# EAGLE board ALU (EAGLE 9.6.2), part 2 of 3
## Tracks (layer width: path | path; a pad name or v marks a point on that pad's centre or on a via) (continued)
GND  (via drill 0.35) (continued)
  Bottom 0.152: v64.14,80.96 64.14,76.84 64.77,76.2 C18.2 65.41,76.2 65.41,70.33 63.82,68.74 63.82,66.67 64.45,66.04 C13.2 64.93,65.88 64.93,61.76 v65.38,61.31 65.09,61.02 C43.2 65.41,55.88 65.41,51.44 66.67,50.16 66.67,47.62 64.77,45.72 64.77,44.77 C46.2 65.09,43.5 63.5,41.91 | 64.14,84.45 64.14,87 | 64.14,87 64.14,87.63 C20.2 64.14,87 | 52.23,43.18 52.23,44.29 C27.2 52.07,44.77 48.1,44.77 47.15,43.82 v45.72,43.82 45.72,48.74 43.18,51.28 v43.18,53.34 46.51,53.34 47.62,54.45 48.74,54.45 50.16,55.88 C62.2 | 52.23,43.18 52.23,38.58 | 52.23,38.58 52.23,33.18 C49.2 | 52.23,43.18 58.42,43.18 | 58.42,43.18 59.69,43.18 60.96,41.91 63.5,41.91 | 52.23,38.58 44.45,30.8 v44.45,30.48 | 58.42,43.18 v58.42,42.55 | 65.09,15.24 C47.2 64.77,21.91 64.77,25.56 66.36,27.15 66.36,30.8 65.41,31.75 65.41,33.02 C48.2 65.09,35.24 66.36,36.51 66.36,39.69 64.14,41.91 63.5,41.91 | 51.12,67.95 C14.2 | C19.2 51.44,87.63 51.44,87.15 49.21,87.15 47.78,85.73 47.78,80.8 51.44,77.15 51.44,76.2 C17.2 51.12,75.56 52.07,74.61 52.07,73.66 51.12,72.71 51.12,67.95 | 37.62,60.01 37.62,66.04 C30.2 | 37.47,55.88 37.47,56.99 36.67,57.79 36.67,59.05 37.62,60.01 | 37.62,60.01 41.91,64.29 v41.91,64.45 41.91,66.04 43.81,67.95 51.12,67.95 | C70.2 51.44,8.89 51.44,10.48 49.85,12.07 49.85,15.24 | C69.2 38.73,8.89 38.73,9.84 39.37,10.48 39.37,11.43 43.18,15.24 | 43.18,15.24 49.85,15.24 | 37.47,55.88 37.47,53.02 35.08,50.64 35.08,47.79 C26.2 38.73,44.45 38.73,42.39 40.16,40.96 40.16,38.26 38.73,36.83 38.73,33.02 C53.2 37.91,32.51 v33.91,32.51 33.91,31.81 38.26,27.46 38.26,21.75 C51.2 38.73,21.59 38.73,19.05 v44.45,19.05 43.18,17.78 43.18,15.24
  Bottom 0.152: 37.47,55.88 C9.2 | 49.85,15.24 v56.52,15.24 65.09,15.24 | C44.2 10.48,40.57 11.68,39.37 v15.24,39.37 10.16,34.29 10.16,33.34 C33.2 10.79,33.02 10.79,31.75 12.06,30.48 13.18,30.48 v15.24,28.42 | v27.94,61.59 v27.94,57.15 | v50.48,22.54 50.48,22.38 51.28,21.59 C50.2 52.07,21.59 49.85,19.37 49.85,15.24 | v80.64,71.75 81.6,72.71 83.5,72.71 v84.45,71.75 | 64.14,84.45 65.09,83.5 65.09,81.92 v64.14,80.96 | v57.15,84.45 57.15,84.3 57.94,83.5 63.18,83.5 64.14,84.45 | v80.64,71.75 81.28,71.12 81.28,69.85 80.01,68.58 80.01,66.52 80.49,66.04 | 124.94,33.97 129.22,33.97 v129.54,34.29 | 23.5,57.31 v24.61,57.31 | v68.58,82.55 68.58,82.07 68.08,81.58 64.75,81.58 v64.14,80.96
ITS  (via drill 0.35)
  Top 0.152: v108.74,44.29 108.84,44.29 109.22,43.92 IC67.2 | v121.28,59.05 121.28,57.79 121.92,57.15 IC62.1
  Route2 0.152: v108.74,44.29 108.74,45.24 113.51,50.01 113.51,50.8 121.28,58.58 v121.28,59.05
LDA  (via drill 0.35)
  Top 0.152: v139.7,35.56 IC55.13 | v115.57,46.36 IC67.8 115.57,48.9 115.76,49.08 v115.76,50.29 | IC68.1 107.95,53.98 109.22,55.25 111.76,55.25 112.24,55.72 114.94,55.72 115.41,55.25 116.51,55.25 v116.53,55.22
  Route2 0.152: v139.7,35.56 128.91,46.36 v115.57,46.36
  Route3 0.152: v116.53,55.22 116.53,51.38 115.76,50.61 v115.76,50.29
LDN  (via drill 0.35)
  Top 0.152: IC68.2 109.22,51.44 109.83,50.82 110.76,50.82 111.26,50.32 v112.42,50.32 | v111.76,44.45 112.71,44.45 113.03,44.13 IC67.5 | v131.13,43.18 138.43,43.18 IC56.1
  Route2 0.152: v131.13,43.18 113.03,43.18 v111.76,44.45
  Route3 0.152: v111.76,44.45 111.76,45.4 112.55,46.2 112.55,50.3 112.53,50.32 v112.42,50.32
MA1  (via drill 0.35)
  Top 0.152: v117.47,66.67 118.11,66.04 118.11,60.01 119.38,58.74 119.38,53.98 118.59,53.18 118.59,37.31 v118.11,36.83 | IC69.2 v109.22,66.36 | IC66.11 111.76,36.2 112.55,35.4 114.78,35.4 v114.94,35.56 | v134.94,71.75 133.03,71.75 131.13,69.85 v128.27,69.85 | IC59.1 v138.43,71.75
  Route2 0.152: v109.22,66.36 109.54,66.67 v117.47,66.67 120.65,69.85 122.24,69.85 123.03,70.64 124.3,70.64 125.09,69.85 v128.27,69.85 | v114.94,35.56 116.2,36.83 v118.11,36.83 | v138.43,71.75 v134.94,71.75
MA2  (via drill 0.35)
  Top 0.152: v110.49,50.16 IC67.12 | IC69.6 v114.3,61.59 | v139.7,77.79 IC59.13
  Route3 0.152: v110.49,50.16 110.49,52.71 115.57,57.79 115.57,60.33 v114.3,61.59
  Route14 0.152: v139.7,77.79 139.22,77.79 128.43,66.99 126.68,66.99 125.25,65.56 125.25,64.29 122.56,61.59 v114.3,61.59
MN1  (via drill 0.35)
  Top 0.152: IC66.4 111.76,29.53 v110.33,28.1 | v107.31,60.96 107.63,60.96 107.95,61.28 IC69.1 | v138.43,86.36 IC60.1
  Route3 0.152: v138.43,86.36 138.43,83.19 127.95,72.71 117,72.71 114.04,69.75 113.57,69.75 107.31,63.5 v107.31,60.96
  Bottom 0.152: v110.33,28.1 110.33,30 106.68,33.66 106.68,51.75 106.05,52.39 106.05,55.88 107.31,57.15 v107.31,60.96
MN2  (via drill 0.35)
  Top 0.152: v114.3,65.41 113.03,64.14 IC69.5 | IC60.13 139.7,91.44 139.06,92.08 137.79,92.08 130.18,84.45 130.18,71.12 129.7,70.64 124.62,70.64 v123.19,69.22 | v108.03,41.42 107.95,41.5 IC67.1
  Route2 0.152: v114.3,65.41 v109.86,60.96
  Route3 0.152: v108.03,41.42 107.98,41.47 107.98,59.08 v109.86,60.96
  Bottom 0.152: v114.3,65.41 114.3,66.2 115.89,67.79 116.84,67.79 116.92,67.87 122.79,67.87 123.19,68.26 v123.19,69.22
MUL/IN/T1/N0  (via drill 0.35)
  Top 0.152: IC31.1 49.53,16.83 49.85,16.51 v52.07,16.51 | v63.18,21.91 62.23,20.95 IC32.1 | v81.28,20.32 IC27.4
  Route14 0.152: v81.28,20.32 81.28,22.38 79.85,23.81 65.09,23.81 v63.18,21.91
  Bottom 0.152: v52.07,16.51 56.04,20.48 56.04,21.43 57.47,22.86 62.23,22.86 v63.18,21.91
MUL/IN/T1/N1  (via drill 0.35)
  Top 0.152: v58.26,24.92 57.15,24.92 IC31.8 | v68.58,22.22 69.85,23.49 IC32.8 | v79.38,20.32 79.69,20.32 82.55,23.18 IC27.10
  Route2 0.152: v58.26,24.92 65.88,24.92 v68.58,22.22
  Bottom 0.152: v79.38,20.32 70.48,20.32 v68.58,22.22
MUL/IN/T1/N2  (via drill 0.35)
  Top 0.152: IC35.1 7.62,17.14 9.37,15.4 10.95,15.4 v12.06,16.51 | v20.32,18.41 21.59,18.41 IC34.1 | v79.38,22.86 80.96,22.86 81.28,23.18 IC27.11
  Route2 0.152: v12.06,16.51 12.38,16.19 18.1,16.19 v20.32,18.41
  Route14 0.152: v79.38,22.86 71.28,22.86 69.61,21.19 65.64,21.19 62.87,18.41 47.15,18.41 45.88,17.14 41.27,17.14 40.01,18.41 v20.32,18.41
MUL/IN/T1/N3  (via drill 0.35)
  Top 0.152: v15.24,22.22 IC35.8 | IC34.8 v29.21,22.22
  Route2 0.152: v15.24,22.22 15.72,22.7 27.17,22.7 27.67,22.2 28.21,22.2 28.23,22.22 v29.21,22.22
MUL/IN/T2/N0  (via drill 0.35)
  Top 0.152: v49.85,20.95 50.8,20 IC31.2 | IC32.2 v63.5,20.95 | IC28.3 80.01,29.21 v78.74,27.94
  Route2 0.152: v49.85,20.95 53.98,20.95 55.4,22.38 61.28,22.38 62.71,20.95 v63.5,20.95 68.58,20.95 75.56,27.94 v78.74,27.94
MUL/IN/T2/N1  (via drill 0.35)
  Top 0.152: IC31.9 55.88,23.23 57.47,21.65 v57.47,21.43 | v81.28,31.75 IC28.4 | v68.58,26.04 IC32.9
  Route3 0.152: v81.28,31.75 80.8,31.27 73.82,31.27 v68.58,26.04 65.09,26.04 v60.64,21.59
  Bottom 0.152: v60.64,21.59 60.48,21.43 v57.47,21.43
MUL/IN/T2/N2  (via drill 0.35)
  Top 0.152: IC35.2 8.89,19.68 v9.53,20.32 | v17.14,17.14 22.7,17.14 22.86,17.3 IC34.2 | IC28.10 82.55,34.92 v83.19,34.29
  Route2 0.152: v9.53,20.32 12.7,17.14 v17.14,17.14
  Route15 0.152: v83.19,34.29 81.92,34.29 78.9,31.27 75.72,31.27 62.87,18.41 47.15,18.41 45.88,17.14 v17.14,17.14
MUL/IN/T2/N3  (via drill 0.35)
  Top 0.152: v13.97,22.86 IC35.9 | v27.94,22.86 IC34.9 | v81.44,37.78 81.44,37.68 81.28,37.52 IC28.11
  Route2 0.152: v13.97,22.86 14.45,23.34 27.46,23.34 v27.94,22.86
  Route3 0.152: v81.44,37.78 81.12,37.78 78.26,34.92 71.91,34.92 70.33,33.34 62.39,33.34 61.44,34.29 58.58,34.29 57.47,35.4 51.59,35.4 51.12,34.92 46.35,34.92 41.91,30.48 35.56,30.48 v27.94,22.86
MUL/IN/T3/N0  (via drill 0.35)
  Top 0.152: v50.8,31.75 50.48,31.75 49.53,30.8 IC36.1 | v62.23,27.94 IC37.1 | IC29.3 80.01,40.64 v78.74,39.37
  Route2 0.152: v78.74,39.37 72.87,39.37 62.23,28.73 v62.23,27.94
  Bottom 0.152: v50.8,31.75 57.15,31.75 60.96,27.94 v62.23,27.94
MUL/IN/T3/N1  (via drill 0.35)
  Top 0.152: v58.42,35.56 57.15,35.56 IC36.8 | v70.8,35.56 69.85,35.56 IC37.8 | v78.74,38.1 80.49,39.85 81.12,39.85 81.28,40.01 IC29.4
  Route3 0.152: v70.8,35.56 v58.42,35.56
  Bottom 0.152: v78.74,38.1 73.34,38.1 v70.8,35.56
MUL/IN/T3/N2  (via drill 0.35)
  Top 0.152: IC39.1 21.59,31.11 21.46,31.24 v21.59,31.37 | v7.62,31.43 IC40.1 | IC29.10 82.55,44.45 v81.28,43.18
  Route2 0.152: v7.62,31.43 7.62,27.94 8.26,27.3 11.43,27.3 15.27,31.15 18.07,31.15 18.8,31.88 21.08,31.88 v21.59,31.37
  Route15 0.152: v81.28,43.18 74.93,36.83 48.42,36.83 47.62,37.62 43.66,37.62 42.23,36.2 23.18,36.2 21.59,34.61 v21.59,31.37
MUL/IN/T3/N3  (via drill 0.35)
  Top 0.152: v19.05,35.56 15.24,35.56 IC40.8 | IC39.8 v29.21,34.61 | IC29.11 81.28,45.09 v79.38,43.18
  Route3 0.152: v19.05,35.56 19.3,35.31 28.51,35.31 v29.21,34.61 44.13,34.61 51.12,41.59 69.22,41.59 70.8,43.18 74.45,43.18 75.56,42.07 78.26,42.07 v79.38,43.18
MUL/IN/T4/N0  (via drill 0.35)
  Top 0.152: v49.53,43.82 IC41.1 | IC42.1 v62.23,42.86 | v80.01,54.29 IC30.3
  Route2 0.152: v62.23,42.86 61.59,43.5 52.23,43.5 51.28,44.45 50.16,44.45 v49.53,43.82
  Route14 0.152: v80.01,54.29 72.07,54.29 62.23,44.45 v62.23,42.86
MUL/IN/T4/N1  (via drill 0.35)
  Top 0.152: v58.58,47.47 57.21,47.47 IC41.8 | v69.53,49.21 69.85,48.9 IC42.8 | IC30.4 81.28,51.59 80.8,51.12 v79.85,51.12
  Route2 0.152: v58.58,47.47 67.79,47.47 v69.53,49.21 71.44,51.12 v79.85,51.12
MUL/IN/T4/N2  (via drill 0.35)
  Top 0.152: IC45.1 7.62,40.01 9.21,38.42 18.41,38.42 20,40.01 v21.59,40.01 IC44.1 | v82.55,57.47 IC30.10
  Route2 0.152: v81.28,50.16 81.12,50.32 71.91,50.32 62.23,40.64 41.12,40.64 40.64,41.12 36.2,41.12 35.72,40.64 22.23,40.64 v21.59,40.01
  Route3 0.152: v82.55,57.47 82.55,55.88 81.28,54.61 v81.28,50.16
MUL/IN/T4/N3  (via drill 0.35)
  Top 0.152: v17.78,47.62 15.24,47.62 IC45.8 | v30.48,47.62 29.21,47.62 IC44.8 | v81.28,60.33 IC30.11
  Route2 0.152: v30.48,47.62 v17.78,47.62
  Route3 0.152: v81.28,60.33 79.38,60.33 70.48,51.44 65.88,51.44 64.29,49.85 61.59,49.85 60.01,51.44 52.55,51.44 50.96,49.85 48.42,49.85 46.83,51.44 34.29,51.44 v30.48,47.62
MUL/OUT/N0  (via drill 0.35)
  Top 0.152: IC27.3 80.01,17.14 v80.64,16.51 | IC50.13 v49.53,88.27
  Route2 0.152: v49.53,88.27 50.16,87.63 50.16,85.73 60.96,74.93 60.96,72.07 63.66,69.37 66.52,69.37 70.17,65.72 70.17,62.87 81.92,51.12 82.87,51.12 85.09,48.9 85.09,37.47 82.15,34.53 82.15,18.02 v80.64,16.51
MUL/OUT/N1  (via drill 0.35)
  Top 0.152: IC33.3 38.1,21.59 v39.37,22.86 | IC50.9 v54.61,87.63
  Route14 0.152: v39.37,22.86 39.37,36.83 44.69,42.15 44.69,60.56 54.61,70.48 54.61,74.93 56.2,76.52 56.2,86.04 v54.61,87.63
MUL/OUT/N2  (via drill 0.35)
  Top 0.152: v38.1,31.43 IC38.3 | IC50.6 v54.61,86.04
  Route14 0.152: v38.1,31.43 38.1,34.29 32.38,40.01 32.38,50.64 32.86,51.12 32.86,52.71 32.38,53.18 32.38,57.47 31.75,58.1 31.75,64.45 33.66,66.36 33.66,67.31 43.97,77.63 43.97,79.85 50.16,86.04 v54.61,86.04
MUL/OUT/N3  (via drill 0.35)
  Top 0.152: IC50.2 v49.53,83.19 | IC43.3 v38.1,40.01
  Route14 0.152: v38.1,40.01 38.1,46.04 39.05,46.99 39.05,60.01 49.85,70.8 49.85,76.84 48.1,78.58 48.1,81.76 v49.53,83.19
MUL/OUT/N4  (via drill 0.35)
  Top 0.152: v46.99,48.26 44.29,45.56 41.75,45.56 39.37,43.18 IC43.4 | v87.63,48.26 87.63,61.59 93.98,67.95 IC51.13
  Route15 0.152: v87.63,48.26 83.82,48.26 82.71,47.15 75.09,47.15 73.98,48.26 v46.99,48.26
MUL/OUT/N5  (via drill 0.35)
  Top 0.152: v94.61,64.77 97.16,67.31 98.61,67.31 99.06,67.75 IC51.9 | IC43.10 40.64,49.37 41.43,50.16 44.45,50.16 v46.99,52.71
  Route3 0.152: v46.99,52.71 57.78,52.71 65.25,60.17 66.2,60.17 67.31,61.28 67.31,62.23 68.58,63.5 80.01,63.5 80.64,64.14 93.98,64.14 v94.61,64.77
MUL/OUT/N6  (via drill 0.35)
  Top 0.152: v39.37,45.72 IC43.11 | IC51.6 v99.06,61.47
  Route3 0.152: v39.37,45.72 48.26,45.72 50.64,48.1 56.67,48.1 56.83,48.26 74.77,48.26 75.41,47.62 82.39,47.62 83.82,49.05 91.73,49.05 97.54,54.86 97.54,61.21 97.79,61.47 v99.06,61.47
MUL/OUT/N7  (via drill 0.35)
  Top 0.152: v25.4,48.9 IC44.11 | v88.9,61.59 93.34,61.59 93.98,62.23 IC51.2
  Route3 0.152: v25.4,48.9 27.3,50.8 29.21,50.8 30.8,52.39 46.04,52.39 46.35,52.07 46.63,51.79 48.93,51.79 49.21,52.07 68.58,52.07 77.31,60.8 80.49,60.8 82.23,62.55 87.95,62.55 v88.9,61.59
MUL/OUT/T1/N0  (via drill 0.35)
  Top 0.152: v49.53,26.99 46.99,26.99 45.4,25.4 45.4,23.81 43.18,21.59 40.96,21.59 39.37,20 IC33.4 | IC36.2 v50.8,28.57 | v61.59,31.75 63.18,31.75 63.5,31.43 IC37.2
  Route2 0.152: v49.53,26.99 50.8,28.26 v50.8,28.57
  Route14 0.152: v61.59,31.75 53.98,31.75 v50.8,28.57
MUL/OUT/T1/N1  (via drill 0.35)
  Top 0.152: IC33.10 40.64,26.04 43.18,28.57 46.35,28.57 v50.8,33.02 | IC36.9 v55.88,34.13 | IC37.9 68.58,37.47 67.63,38.42 v65.25,38.42
  Route2 0.152: v50.8,33.02 54.77,33.02 v55.88,34.13
  Bottom 0.152: v65.25,38.42 65.09,38.42 60.64,33.97 56.04,33.97 v55.88,34.13
MUL/OUT/T1/N2  (via drill 0.35)
  Top 0.152: IC39.2 v22.86,28.57 | IC33.11 39.37,25.4 v37.47,27.3 | IC40.2 v8.89,28.57
  Route2 0.152: v37.47,27.3 34.29,27.3 33.02,28.57 28.89,28.57 27.94,29.53 25.72,29.53 24.77,28.57 v22.86,28.57
  Route14 0.152: v22.86,28.57 22.83,28.6 19.37,28.6 17.81,30.16 10.48,30.16 v8.89,28.57
MUL/OUT/T1/N3  (via drill 0.35)
  Top 0.152: IC34.11 v25.4,26.04 | v13.97,34.61 IC40.9 | v27.94,34.61 IC39.9
  Route14 0.152: v13.97,34.61 20.32,34.61 21.27,35.56 26.99,35.56 v27.94,34.61 28.89,33.66 28.89,28.26 26.67,26.04 v25.4,26.04
MUL/OUT/T2/N0  (via drill 0.35)
  Top 0.152: v47.94,33.02 40.96,33.02 39.37,31.43 IC38.4 | IC41.2 v50.8,38.1 | v63.5,40.01 IC42.2
  Route2 0.152: v63.5,40.01 60.33,36.83 57.31,36.83 56.67,36.2 52.7,36.2 v50.8,38.1 50.8,35.88 v47.94,33.02
MUL/OUT/T2/N1  (via drill 0.35)
  Top 0.152: v48.26,46.99 47.62,46.36 47.62,42.23 44.77,39.37 42.23,39.37 40.64,37.78 IC38.10 | IC41.9 v55.88,49.53 | IC42.9 68.58,48.26 66.99,49.85 v65.88,49.85
  Route2 0.152: v48.26,46.99 49.53,48.26 54.61,48.26 v55.88,49.53
  Bottom 0.152: v65.88,49.85 62.71,46.67 58.1,46.67 55.88,48.9 v55.88,49.53
MUL/OUT/T2/N2  (via drill 0.35)
  Top 0.152: v8.89,42.8 IC45.2 | IC44.2 v22.86,38.1 | v39.37,38.73 IC38.11
  Route2 0.152: v8.89,42.8 9.27,42.8 13.97,38.1 21.3,38.1 21.32,38.08 21.86,38.08 21.89,38.1 v22.86,38.1 24.13,39.37 25.88,39.37 26.51,38.73 v39.37,38.73
MUL/OUT/T2/N3  (via drill 0.35)
  Top 0.152: v13.97,46.04 IC45.9 | IC44.9 v27.94,45.09 | IC39.11 25.4,37.08 27.3,38.99 v27.3,39.69
  Route2 0.152: v13.97,46.04 14.95,45.06 16.46,45.06 16.49,45.09 v27.94,45.09
  Route14 0.152: v27.3,39.69 26.19,40.8 26.19,43.34 v27.94,45.09
N$1  (via drill 0.35)
  Top 0.152: v81.92,74.45 IC1.5 | v113.03,81.92 113.03,81.53 112.39,80.9 IC2.12
  Route2 0.152: v81.92,74.45 81.92,77.47 83.82,79.38 86.36,81.92 92.39,81.92 94.3,83.82 99.54,83.82 101.44,81.92 109.08,81.92 109.58,82.41 110.13,82.41 110.63,81.92 v113.03,81.92
N$2  (via drill 0.35)
  Top 0.152: IC7.13 111.12,89.15 109.86,87.88 IC7.3 v109.86,81.76 | v96.52,31.75 IC10.4 | v93.98,44.45 93.98,50.16 94.61,50.8 IC5.3 94.61,53.34 95.89,54.61 IC5.13
  Route3 0.152: v96.52,31.75 96.52,41.91 95.25,43.18 | v93.98,44.45 95.25,43.18 | v109.86,81.76 111.92,81.76 113.19,80.49 115.89,80.49 120.33,76.04 120.33,75.09 118.52,73.28 113.92,73.28 110.49,69.85 108.9,69.85 107.63,68.58 107.63,66.99 100.97,60.33 100.97,48.9 95.25,43.18
N$3  (via drill 0.35)
  Top 0.152: IC1.13 80.64,77.47 79.38,76.2 IC1.3 v79.38,71.75 | IC10.3 95.25,28.89 96.2,27.94 v96.52,27.94 | IC3.3 94.61,43.18 95.89,44.45 IC3.13 v95.89,45.97
  Route14 0.152: v79.38,71.75 79.38,71.12 79.06,70.8 79.06,68.9 89.53,58.42 89.53,52.68 89.72,52.5 89.72,51.16 89.53,50.98 89.53,46.74 | 89.53,46.74 89.53,34.92 91.44,33.02 91.44,31.11 93.19,29.37 94.77,29.37 96.2,27.94 v96.52,27.94 | v89.44,46.74 89.53,46.74
  Route15 0.152: v95.89,45.97 93.98,45.97 93.22,46.74 v89.44,46.74
N$4  (via drill 0.35)
  Top 0.152: v83.19,77.47 IC1.11 | v102.87,78.11 103.35,77.63 108.11,77.63 108.58,78.11 IC2.15
  Route2 0.152: v102.87,78.11 102.71,78.11 101.6,79.22 84.93,79.22 v83.19,77.47
N$5  (via drill 0.35)
  Top 0.152: v100.33,43.18 97.79,43.18 97.16,42.55 IC3.5 | v130.65,27.3 135.1,22.86 135.1,17.94 135.89,17.14 138.75,17.14 139.06,17.46 IC4.2
  Route2 0.152: v100.33,43.18 104.14,43.18 107,40.32 108.9,40.32 109.62,39.61 109.62,38.18 115.65,32.15 117.08,32.15 121.92,27.3 v130.65,27.3
N$6  (via drill 0.35)
  Top 0.152: v89.38,90.81 85.09,90.81 IC6.8 | v102.23,90.81 107.31,85.73 IC7.1
  Route2 0.152: v102.23,90.81 v89.38,90.81
N$7  (via drill 0.35)
  Top 0.152: v82.55,85.88 IC6.5 | IC7.15 108.58,92.08 107.95,92.71 106.68,92.71 v105.25,91.28
  Route3 0.152: v105.25,91.28 103.5,89.53 92.71,89.53 89.06,85.88 v82.55,85.88
N$8  (via drill 0.35)
  Top 0.152: IC3.11 98.42,46.04 98.74,45.72 v99.06,45.72 | v138.43,23.49 141.6,20.32 IC4.4
  Route14 0.152: v99.06,45.72 111.76,45.72 114.46,43.02 122.08,43.02 122.56,42.55 127.48,42.55 128.35,41.67 128.35,36.75 138.43,26.67 v138.43,23.49
N$9  (via drill 0.35)
  Top 0.152: IC5.5 97.16,51.44 v97.79,50.8 | IC2.6 113.67,71.18 v113.32,70.83
  Route14 0.152: v113.32,70.83 111.32,68.83 108.2,68.83 105.06,65.69 v105.06,60.96
  Bottom 0.152: v97.79,50.8 98.42,51.44 104.01,51.44 105.06,52.48 v105.06,60.96
N$10  (via drill 0.35)
  Top 0.152: v92.08,54.61 IC5.1 | IC6.1 v77.47,81.28
  Route14 0.152: v86.36,69.22 86.36,73.03 78.11,81.28 v77.47,81.28
  Bottom 0.152: v92.08,54.61 92.08,63.5 v86.36,69.22
N$11  (via drill 0.35)
  Top 0.152: IC5.15 93.34,57.59 v93.31,57.56 | IC6.12 v80.01,89.22
  Route15 0.152: v80.01,89.22 80.01,84.14 82.23,81.92 v83.19,81.92
  Bottom 0.152: v93.31,57.56 92.88,58 92.88,68.74 92.41,69.21 92.41,71.93 83.19,81.15 v83.19,81.92
N$12  (via drill 0.35)
  Top 0.152: IC2.10 v114.94,75.56 | IC5.11 v98.42,60.45
  Route2 0.152: v114.94,75.56 114.94,74.93 113.86,73.85 111.76,73.85 109.98,72.07 108.9,72.07 v106.68,69.85 | v103.89,67.06 100.58,67.06 97.63,64.1 97.63,61.25 v98.42,60.45
  Route3 0.152: v106.68,69.85 v103.89,67.06
N$13  (via drill 0.35)
  Top 0.152: IC2.2 108.58,74.52 v108.54,74.56 | IC7.5 112.39,82.55 110.49,80.64 108.9,80.64 v108.58,80.96
  Bottom 0.152: v108.58,80.96 108.86,80.69 108.86,74.88 v108.54,74.56
N$14  (via drill 0.35)
  Top 0.152: IC70.5 97.79,17.14 95.89,15.24 v90.17,15.24
  Bottom 0.152: REGISTER/OUT.4 v90.17,15.24
N$15
  Top 0.152: IC26.11 67.94,76.2 68.74,75.41 70.96,75.41 71.75,76.2 71.75,86.68 69.69,88.74 65.25,88.74 64.77,89.22 IC9.11
N$16  (via drill 0.35)
  Top 0.152: IC2.4 111.12,74.3 v111.76,74.93 | v111.92,86.2 111.92,87.15 113.67,88.9 IC7.11
  Bottom 0.152: v111.92,86.2 112.55,85.57 112.55,82.71 111.76,81.92 v111.76,74.93
N$17  (via drill 0.35)
  Top 0.152: v55.24,54.61 53.66,54.61 53.34,54.29 IC16.5 | v64.45,54.45 64.45,54.39 64.77,54.08 IC17.3 64.77,52.07 65.41,51.44 66.67,51.44 67.31,52.07 IC17.5
  Route2 0.152: v55.24,54.61 56.04,55.4 63.5,55.4 v64.45,54.45
N$18  (via drill 0.35)
  Top 0.152: IC18.1 34.29,54.13 33.66,54.77 33.66,55.88 v34.92,57.15 | IC16.3 v50.8,54.29
  Route2 0.152: v50.8,54.29 50.8,53.34 50.16,52.71 48.26,52.71 42.55,58.42 36.2,58.42 v34.92,57.15
N$19  (via drill 0.35)
  Top 0.152: v100.33,22.22 IC70.8
  Route2 0.152: REGISTER/OUT.3 84.45,6.35 95.89,17.78 99.06,17.78 100.33,19.05 v100.33,22.22
N$20  (via drill 0.35)
  Top 0.152: v84.45,65.41 83.5,65.41 82.55,64.45 IC8.5 | v90.81,20.32 v90.81,36.83
  Bottom 0.152: v90.81,36.83 90.81,42.07 90.33,42.55 90.33,44.45 90.81,44.93 90.81,52.07 86.36,56.52 86.36,63.5 v84.45,65.41 | v90.81,20.32 91.6,19.53 91.6,11.59 REGISTER/OUT.2
N$21
  Top 0.152: IC12.5 53.34,4.45 55.88,1.91 63.5,1.91 64.77,3.17 | IC11.3 64.77,3.17 | IC11.5 67.31,4.45 66.04,3.17 64.77,3.17
N$22  (via drill 0.35)
  Top 0.152: v87,36.83 86.84,36.99 86.84,64.93 v87,65.09 | IC8.12 v80.01,70.48
  Route3 0.152: v87,36.83 87,8.26 REGISTER/OUT.1 | v80.01,70.48 81.6,70.48 v87,65.09
N$25
  Top 0.152: IC13.1 35.56,4.13 37.15,2.54 50.16,2.54 50.8,3.17 IC12.3
N$29  (via drill 0.35)
  Top 0.152: IC13.2 v36.83,4.43 | v52.07,4.45 IC12.4
  Route3 0.152: v36.83,4.43 38.4,2.86 50.8,2.86 52.07,4.13 v52.07,4.45
N$30  (via drill 0.35)
  Top 0.152: v45.72,56.52 45.09,55.88 38.1,55.88 35.56,53.34 IC18.2 | v53.98,49.53 53.98,50.16 52.07,52.07 IC16.4
  Route14 0.152: v45.72,56.52 51.44,50.8 52.7,50.8 v53.98,49.53
N$31  (via drill 0.35)
  Top 0.152: v49.53,10.16 IC12.13 | v66.04,4.45 IC11.4 66.04,6.98 63.5,9.53 IC11.13
  Bottom 0.152: v49.53,10.16 49.53,8.26 53.98,3.81 65.41,3.81 v66.04,4.45
N$32  (via drill 0.35)
  Top 0.152: v49.53,57.15 IC16.13 | IC17.13 63.5,56.52 v62.87,56.52 64.14,56.52 66.04,54.61 IC17.4
  Route2 0.152: v49.53,57.15 50.48,56.2 62.55,56.2 v62.87,56.52
N$33  (via drill 0.35)
  Top 0.152: v18.57,55.09 18.41,54.93 17.46,54.93 17.14,54.61 14.61,54.61 13.97,53.98 IC20.6 | IC19.6 v26.67,55.25 | v66.04,57.15 IC17.11
  Route2 0.152: v26.67,55.25 26.04,54.61 19.05,54.61 v18.57,55.09
  Route15 0.152: v66.04,57.15 65.56,57.63 55.72,57.63 55.17,57.07 55.17,56.28 52.39,53.5 47.31,53.5 44.93,55.88 27.3,55.88 v26.67,55.25
N$38  (via drill 0.35)
  Top 0.152: v50.8,60.96 IC16.12 | 64.77,60.64 63.82,60.64 v63.5,60.96 | IC17.12 64.77,60.64 | IC17.10 67.31,60.33 66.99,60.64 64.77,60.64
  Bottom 0.152: v50.8,60.96 51.12,61.28 63.18,61.28 v63.5,60.96
N$39  (via drill 0.35)
  Top 0.152: IC15.6 13.97,3.81 14.76,3.02 v19.68,3.02 | v23.5,3.02 26.19,3.02 27.94,4.76 IC14.6 | v66.04,10.16 IC11.11
  Route2 0.152: v19.68,3.02 v23.5,3.02 23.81,3.33 47.15,3.33 47.94,2.54 59.37,2.54 66.04,9.21 v66.04,10.16
N$40  (via drill 0.35)
  Top 0.152: v50.8,13.34 IC12.12 | IC11.12 64.77,13.65 65.09,13.97 v66.04,13.97 66.99,13.97 67.31,13.65 IC11.10
  Route2 0.152: v50.8,13.34 50.8,12.22 51.28,11.75 63.82,11.75 v66.04,13.97
N$41
  Top 0.152: IC13.5 40.64,7.62 42.07,9.05 51.91,9.05 53.34,10.48 IC12.10
N$42  (via drill 0.35)
  Top 0.152: IC12.11 v52.07,13.34 | v41.91,4.45 IC13.6
  Route3 0.152: v52.07,13.34 50.48,11.75 49.21,11.75 v41.91,4.45
N$43  (via drill 0.35)
  Top 0.152: v48.26,55.25 48.1,55.4 40.16,55.4 39.37,54.61 IC18.5 | v52.07,54.61 52.07,56.2 53.34,57.47 IC16.10
  Route2 0.152: v48.26,55.25 51.44,55.25 v52.07,54.61
N$44  (via drill 0.35)
  Top 0.152: v41.91,54.61 41.27,54.61 40.64,53.98 IC18.6 | v52.07,57.47 IC16.11
  Bottom 0.152: v52.07,57.47 51.44,58.1 46.04,58.1 45.4,58.1 v41.91,54.61
N$45  (via drill 0.35)
  Top 0.152: IC19.5 25.4,51.44 25.37,51.41 v22.92,51.41 22.86,51.41 IC19.3 | v13.97,50.16 12.7,51.44 IC20.5
  Route2 0.152: v13.97,50.16 14.92,49.21 20.73,49.21 v22.92,51.41
N$46  (via drill 0.35)
  Top 0.152: v8.89,57.47 IC20.13 | IC19.4 24.13,53.98 v21.59,56.52 IC19.13
  Route2 0.152: v8.89,57.47 9.84,56.52 13.52,56.52 13.7,56.7 18.57,56.7 18.78,56.49 19.32,56.49 19.34,56.52 v21.59,56.52
N$47  (via drill 0.35)
  Top 0.152: IC20.4 11.43,50.8 13.34,48.9 14.13,48.9 v18.57,53.34 | v34.92,54.61 36.83,56.52 39.69,56.52 40.64,57.47 IC18.9
  Route2 0.152: v18.57,53.34 33.66,53.34 v34.92,54.61
N$48
  Top 0.152: IC15.5 12.7,3.17 13.97,1.91 20.95,1.91 23.18,4.13 24.13,4.13 | IC14.3 24.13,4.13 | IC14.5 26.67,4.45 26.35,4.13 24.13,4.13
N$49
  Top 0.152: 22.86,9.37 10.95,9.37 8.89,11.43 IC15.13 | IC14.13 22.86,9.37 | 22.86,9.37 25.4,6.83 IC14.4
N$50  (via drill 0.35)
  Top 0.152: IC15.4 11.43,6.98 12.7,8.26 v22.86,8.26 | IC13.9 v41.91,10.48
  Route2 0.152: v41.91,10.48 40.32,8.89 36.51,8.89 35.24,7.62 23.5,7.62 v22.86,8.26
N$51  (via drill 0.35)
  Top 0.152: v10.16,6.98 IC15.3 | v43.18,13.34 IC13.8
  Route2 0.152: v10.16,6.98 10.32,7.14 33.5,7.14 34.29,6.35 41.91,6.35 43.18,7.62 v43.18,13.34
N$52  (via drill 0.35)
  Top 0.152: v10.16,54.29 IC20.3 | IC18.8 v41.91,57.47
  Route2 0.152: v41.91,57.47 39.85,55.4 29.21,55.4 27.8,54 18.3,54 16.99,52.68 11.77,52.68 v10.16,54.29
N$53  (via drill 0.35)
  Top 0.152: IC20.12 10.16,60.33 10.79,60.96 v13.34,60.96 | IC19.12 22.86,60.48 | IC19.10 25.4,60.33 25.24,60.48 22.86,60.48 | 22.86,60.48 22.38,60.96 v21.59,60.96
  Route2 0.152: v21.59,60.96 21.15,60.52 18.69,60.52 18.26,60.96 v13.34,60.96
N$54
  Top 0.152: IC15.12 10.16,13.34 11.91,15.08 22.38,15.08 24.13,13.34 IC14.12 24.13,10.48 24.45,10.16 26.35,10.16 26.67,10.48 IC14.10
N$55  (via drill 0.35)
  Top 0.152: IC15.10 12.7,13.34 13.34,13.97 v21.59,13.97 | v38.1,10.48 IC13.12
  Route2 0.152: v38.1,10.48 36.43,12.14 23.57,12.14 21.75,13.97 v21.59,13.97
N$56  (via drill 0.35)
  Top 0.152: v21.91,10.16 12.06,10.16 11.43,10.79 IC15.11 | v36.83,10.48 IC13.13
  Route2 0.152: v36.83,10.48 36.51,10.16 v21.91,10.16
N$57  (via drill 0.35)
  Top 0.152: v13.97,56.04 13.81,56.04 12.7,57.15 IC20.10 | v36.2,57.15 36.2,57.79 36.83,58.42 IC18.12
  Route2 0.152: v36.2,57.15 34.92,55.88 27.78,55.88 27.15,56.52 25.56,56.52 24.13,55.09 20.95,55.09 20,56.04 v13.97,56.04
N$58  (via drill 0.35)
  Top 0.152: v11.43,57.47 IC20.11 | IC18.13 v35.56,60.96
  Route2 0.152: v11.43,57.47 14.29,57.47 16.99,60.17 24.29,60.17 25.4,59.05 27.3,59.05 29.21,60.96 v35.56,60.96
N$59  (via drill 0.35)
  Top 0.152: IC21.5 53.34,64.14 v53.98,64.77 | 64.45,64.77 64.77,64.45 IC22.3 | 64.45,64.77 v63.5,64.77 | 64.45,64.77 65.11,65.43 66.31,65.43 67.31,64.43 IC22.5
  Route2 0.152: v63.5,64.77 v53.98,64.77
N$60  (via drill 0.35)
  Top 0.152: v47.15,66.67 46.99,66.83 36.67,66.83 34.29,64.45 IC23.1 | v49.21,66.67 50.8,65.09 IC21.3
  Route2 0.152: v49.21,66.67 v47.15,66.67
N$61  (via drill 0.35)
  Top 0.152: v43.66,66.04 37.15,66.04 35.56,64.45 IC23.2 | v60.33,60.33 59.69,60.96 52.7,60.96 52.07,61.59 IC21.4
  Bottom 0.152: v60.33,60.33 60.01,60.64 53.66,60.64 52.86,59.85 49.85,59.85 v43.66,66.04
N$62  (via drill 0.35)
  Top 0.152: IC21.13 49.53,67.31 v52.07,64.77 | v62.87,66.67 62.87,67.95 63.5,68.58 IC22.13 | v66.04,64.77 IC22.4
  Route2 0.152: v52.07,64.77 53.34,66.04 62.23,66.04 v62.87,66.67 64.14,66.67 v66.04,64.77
N$63  (via drill 0.35)
  Top 0.152: IC25.6 13.97,62.23 14.61,61.59 v19.05,61.59 | v26.67,64.45 IC24.6 | v66.04,67.31 IC22.11
  Route2 0.152: v66.04,67.31 66.99,66.36 66.99,64.45 66.04,63.5 60.48,63.5 59.85,64.14 56.04,64.14 55.4,63.5 29.84,63.5 28.89,64.45 v26.67,64.45 23.34,64.45 20.48,61.59 v19.05,61.59
N$64  (via drill 0.35)
  Top 0.152: v53.98,67.31 51.75,67.31 50.8,68.26 IC21.12 | IC22.12 v64.77,67.63 64.77,66.67 65.41,66.04 66.04,66.04 67.31,67.31 IC22.10
  Route2 0.152: v64.77,67.63 54.29,67.63 v53.98,67.31
N$65  (via drill 0.35)
  Top 0.152: IC23.5 39.37,64.77 39.85,65.25 45.56,65.25 v45.72,65.41 | IC21.10 v53.34,70.48
  Route15 0.152: v53.34,70.48 53.34,68.58 50.16,65.41 v45.72,65.41
N$66  (via drill 0.35)
  Top 0.152: v40.64,64.45 IC23.6 | IC21.11 v52.07,70.48
  Route2 0.152: v40.64,64.45 40.64,64.77 43.81,67.95 46.99,67.95 49.53,70.48 v52.07,70.48
N$67  (via drill 0.35)
  Top 0.152: v13.97,64.77 13.34,64.77 12.7,64.14 IC25.5 | 22.86,64.77 v21.59,66.04 | IC24.3 22.86,64.77 | 22.86,64.77 24.77,64.77 25.4,64.14 IC24.5
  Bottom 0.152: v13.97,64.77 20.32,64.77 v21.59,66.04
N$68  (via drill 0.35)
  Top 0.152: v13.34,67.31 12.7,66.67 10.16,66.67 8.89,67.95 IC25.13 | v17.78,67.31 17.78,68.58 19.68,70.48 20.95,70.48 21.59,69.85 IC24.13 | v24.13,61.59 IC24.4
  Route2 0.152: v17.78,67.31 v13.34,67.31
  Route14 0.152: v17.78,67.31 17.78,65.56 21.11,62.23 23.5,62.23 v24.13,61.59
N$69  (via drill 0.35)
  Top 0.152: v11.43,64.77 IC25.4 | v29.84,73.98 37.47,73.98 40.64,70.8 IC23.9
  Route14 0.152: v11.43,64.77 12.54,64.77 21.75,73.98 v29.84,73.98
N$70  (via drill 0.35)
  Top 0.152: IC25.3 10.16,65.41 v8.89,66.67 | v22.86,80.64 31.75,80.64 41.91,70.48 IC23.8
  Route3 0.152: v8.89,66.67 8.89,71.75 10.16,73.03 15.88,73.03 22.86,80.01 v22.86,80.64
N$71  (via drill 0.35)
  Top 0.152: v10.16,67.63 IC25.12 | IC24.12 v22.86,67.63 25.4,67.63 IC24.10
  Route2 0.152: v22.86,67.63 20.64,67.63 16.83,63.82 10.95,63.82 10.16,64.61 v10.16,67.63
N$72  (via drill 0.35)
  Top 0.152: IC25.10 12.7,70.48 13.34,71.12 v13.97,71.12 | IC23.12 v36.83,71.44
  Bottom 0.152: v13.97,71.12 15.24,72.39 35.88,72.39 v36.83,71.44
N$73  (via drill 0.35)
  Top 0.152: v11.75,70.8 11.69,70.8 11.43,70.54 IC25.11 | IC23.13 v35.56,71.12
  Route2 0.152: v35.56,71.12 35.24,71.44 16.83,71.44 15.24,69.85 12.7,69.85 v11.75,70.8
N$74  (via drill 0.35)
  Top 0.152: v54.61,16.51 IC31.5 | v62.87,16.51 63.5,16.51 64.14,17.14 | 64.14,17.14 64.77,17.78 IC32.3 | IC32.5 67.31,17.78 66.67,17.14 64.14,17.14
  Bottom 0.152: v62.87,16.51 v54.61,16.51
N$75  (via drill 0.35)
  Top 0.152: IC33.1 35.56,16.83 37.15,15.24 45.56,15.24 v46.67,16.35 | v52.07,20 IC31.3
  Route2 0.152: v46.67,16.35 50.32,20 v52.07,20
N$76  (via drill 0.35)
  Top 0.152: IC33.2 36.83,17.14 37.94,16.03 v40.32,16.03 | IC31.4 v53.34,20
  Route3 0.152: v40.32,16.03 41.12,15.24 48.58,15.24 v53.34,20
N$77  (via drill 0.35)
  Top 0.152: v57.78,20.32 54.61,20.32 50.8,24.13 IC31.13 | IC32.4 v66.04,20 66.04,20.95 63.5,23.49 IC32.13
  Route2 0.152: v66.04,20 61.28,20 60.96,20.32 v57.78,20.32
N$78  (via drill 0.35)
  Top 0.152: v13.97,20.95 IC35.6 | IC34.6 v27.94,20 | v66.04,22.86 IC32.11
  Route2 0.152: v13.97,20.95 21.75,20.95 22.7,20 v27.94,20
  Route15 0.152: v66.04,22.86 54.61,22.86 53.34,21.59 50.51,21.59 49.87,22.22 49.37,22.22 48.74,21.59 29.53,21.59 v27.94,20
N$79  (via drill 0.35)
  Top 0.152: v52.07,26.67 IC31.12 | v62.87,26.67 63.5,26.67 64.14,26.04 64.77,26.04 | IC32.10 67.31,25.4 66.67,26.04 64.77,26.04 | IC32.12 64.77,26.04
  Bottom 0.152: v62.87,26.67 v52.07,26.67
N$80
  Top 0.152: IC31.10 54.61,25.4 52.55,27.46 51.59,27.46 50.32,26.19 47.78,26.19 47.31,25.72 47.31,24.76 43.5,20.95 41.59,20.95 40.64,20 IC33.5
N$81  (via drill 0.35)
  Top 0.152: IC31.11 v53.34,23.18 | IC33.6 41.91,19.68 42.55,20.32 44.13,20.32 48.26,24.45 v48.26,25.4
  Route2 0.152: v48.26,25.4 51.12,25.4 v53.34,23.18
N$82
  Top 0.152: IC35.5 12.7,16.99 13.49,16.19 24.13,16.19 | IC34.3 24.13,16.19 | IC34.5 26.67,17.3 25.56,16.19 24.13,16.19
N$83  (via drill 0.35)
  Top 0.152: IC35.13 v8.89,23.49 | IC34.4 25.4,20 23.81,21.59 v22.86,21.59 IC34.13
  Route3 0.152: v8.89,23.49 9.84,24.45 17.14,24.45 20,21.59 v22.86,21.59
N$84  (via drill 0.35)
  Top 0.152: v11.43,20.32 IC35.4 | IC33.9 v41.91,26.04
  Route2 0.152: v41.91,26.04 41.91,24.13 36.35,18.57 21.75,18.57 20.02,20.3 13.7,20.3 13.68,20.32 v11.43,20.32
N$85  (via drill 0.35)
  Top 0.152: v10.16,16.51 IC35.3 | v43.18,23.18 IC33.8
  Route2 0.152: v10.16,16.51 11.59,15.08 21.27,15.08 23.34,17.14 37.15,17.14 v43.18,23.18
N$86  (via drill 0.35)
  Top 0.152: v10.16,26.04 IC35.12 | v17.14,27.3 22.86,27.3 24.13,26.04 IC34.12 24.13,23.49 24.77,22.86 26.04,22.86 26.67,23.49 IC34.10
  Route3 0.152: v17.14,27.3 14.45,27.3 13.81,27.94 12.06,27.94 v10.16,26.04
N$87  (via drill 0.35)
  Top 0.152: v36.2,22.86 37.78,22.86 38.1,23.18 IC33.12 | v12.7,23.18 IC35.10
  Route2 0.152: v12.7,23.18 14.31,24.79 20.59,24.79 20.61,24.76 34.29,24.76 v36.2,22.86
N$88  (via drill 0.35)
  Top 0.152: IC35.11 v11.43,26.04 | IC33.13 v36.83,26.04
  Route14 0.152: v36.83,26.04 35.59,24.79 24.51,24.79 23.78,25.53 11.94,25.53 v11.43,26.04
N$89  (via drill 0.35)
  Top 0.152: v54.61,28.57 IC36.5 | IC37.5 67.31,27.94 66.67,27.3 v64.77,27.3 IC37.3
  Route2 0.152: v54.61,28.57 55.88,27.3 60.17,27.3 61.91,25.56 63.82,25.56 64.77,26.51 v64.77,27.3
N$90  (via drill 0.35)
  Top 0.152: IC36.3 v52.07,28.57 | v35.56,31.43 IC38.1
  Route2 0.152: v35.56,31.43 35.88,31.43 36.83,32.38 37.15,32.38 40.64,32.38 41.59,31.43 49.21,31.43 v52.07,28.57
N$91  (via drill 0.35)
  Top 0.152: IC38.2 36.83,29.21 38.1,27.94 v40.64,27.94 | v59.05,28.57 59.05,29.84 57.15,31.75 53.66,31.75 53.34,31.43 IC36.4
  Bottom 0.152: v40.64,27.94 47.94,27.94 50.48,30.48 57.15,30.48 v59.05,28.57
N$92  (via drill 0.35)
  Top 0.152: v59.05,33.02 53.34,33.02 50.8,35.56 IC36.13 | IC37.4 66.04,31.75 65.41,32.38 64.14,32.38 63.5,33.02 v63.5,34.61 IC37.13
  Route2 0.152: v63.5,34.61 61.91,33.02 v59.05,33.02
N$93  (via drill 0.35)
  Top 0.152: IC40.6 13.97,31.11 15.24,32.38 17.78,32.38 v19.37,30.8 | v27.94,31.43 IC39.6 | v66.04,34.61 IC37.11
  Route2 0.152: v19.37,30.8 20.07,30.1 25.81,30.1 27.15,31.43 v27.94,31.43
  Route15 0.152: v66.04,34.61 62.23,30.8 50.16,30.8 48.26,28.89 35.88,28.89 33.34,31.43 v27.94,31.43
N$94  (via drill 0.35)
  Top 0.152: IC36.12 52.07,36.83 v53.34,38.1 | v63.5,38.1 64.14,37.47 64.77,37.47 | IC37.12 64.77,37.47 | IC37.10 67.31,37.15 66.99,37.47 64.77,37.47
  Bottom 0.152: v63.5,38.1 63.02,38.58 53.82,38.58 v53.34,38.1
N$95  (via drill 0.35)
  Top 0.152: v42.55,32.23 41.43,32.23 40.64,31.43 IC38.5 | IC36.10 v54.61,37.47
  Route2 0.152: v42.55,32.23 50.01,39.69 53.34,39.69 54.61,38.42 v54.61,37.47
N$96  (via drill 0.35)
  Top 0.152: v50.64,34.13 50.48,34.13 48.42,32.07 43.5,32.07 41.91,30.48 IC38.6 | IC36.11 v53.34,34.29
  Route2 0.152: v53.34,34.29 53.18,34.13 v50.64,34.13
N$97  (via drill 0.35)
  Top 0.152: v12.7,26.67 IC40.5 | IC39.3 v24.13,27.3 | v26.67,28.57 IC39.5
  Route3 0.152: v24.13,27.3 26.04,27.3 26.67,27.94 v26.67,28.57
  Bottom 0.152: v12.7,26.67 13.18,26.19 23.02,26.19 v24.13,27.3
N$98  (via drill 0.35)
  Top 0.152: IC39.13 v22.86,34.29 25.4,31.75 IC39.4 | v8.89,34.61 IC40.13
  Route14 0.152: v22.86,34.29 22.23,33.66 9.84,33.66 v8.89,34.61
N$99  (via drill 0.35)
  Top 0.152: v11.43,28.57 IC40.4 | v36.2,33.66 40.01,33.66 41.91,35.56 IC38.9
  Route2 0.152: v36.2,33.66 30.64,33.66 29.88,32.89 18.92,32.89 17.78,31.75 14.61,31.75 v11.43,28.57
N$100  (via drill 0.35)
  Top 0.152: v10.16,31.43 IC40.3 | v44.45,36.2 43.18,36.2 IC38.8
  Route2 0.152: v10.16,31.43 11.75,33.02 17.78,33.02 18.41,33.66 20.95,36.2 34.04,36.2 v44.45,36.2
N$101  (via drill 0.35)
  Top 0.152: v10.16,37.62 IC40.12 | v24.26,38.1 24.13,37.97 IC39.12 24.13,34.8 24.64,34.29 26.16,34.29 26.67,34.8 IC39.10
  Route15 0.152: v24.26,38.1 22.67,36.51 20,36.51 18.41,38.1 10.64,38.1 v10.16,37.62
N$102  (via drill 0.35)
  Top 0.152: IC40.10 12.7,37.47 13.02,37.78 16.83,37.78 v17.78,36.83 | IC38.12 v38.1,37.78
  Route2 0.152: v17.78,36.83 37.15,36.83 v38.1,37.78
N$103  (via drill 0.35)
  Top 0.152: v11.43,34.61 IC40.11 | IC38.13 v36.83,37.78
  Route2 0.152: v11.43,34.61 11.43,35.56 13.49,37.62 18.89,37.62 19.33,37.19 36.23,37.19 v36.83,37.78
N$104  (via drill 0.35)
  Top 0.152: v57.15,44.45 56.2,44.45 54.61,42.86 IC41.5 | v63.5,44.45 63.5,43.18 64.77,41.91 IC42.3 64.77,40.64 65.41,40.01 66.67,40.01 67.31,40.64 IC42.5
  Bottom 0.152: v63.5,44.45 v57.15,44.45
N$105  (via drill 0.35)
  Top 0.152: v35.56,43.18 IC43.1 | v50.8,43.18 51.44,43.18 52.07,42.55 IC41.3
  Route2 0.152: v50.8,43.18 49.21,41.59 37.15,41.59 v35.56,43.18
N$106  (via drill 0.35)
  Top 0.152: v120.02,84.45 120.02,83.82 122.24,81.6 124.46,81.6 125.73,80.33 IC53.4 | v52.07,80.64 IC49.11
  Route3 0.152: v120.02,84.45 119.54,84.45 81.44,84.45 81.16,84.73 78.54,84.73 78.26,84.45 63.5,84.45 63.02,83.98 59.53,83.98 v58.42,85.09
  Route15 0.152: v52.07,80.64 55.24,80.64 58.42,83.82 v58.42,85.09
N$107  (via drill 0.35)
  Top 0.152: v36.83,44.13 IC43.2 | IC41.4 53.34,42.55 51.44,44.45 50.8,44.45 v49.53,45.72
  Route2 0.152: v36.83,44.13 41.59,44.13 43.18,45.72 v49.53,45.72
N$108  (via drill 0.35)
  Top 0.152: v50.8,45.72 IC41.13 | v63.5,49.05 IC42.13 63.5,45.72 66.04,43.18 IC42.4
  Route2 0.152: v50.8,45.72 53.98,45.72 57.31,49.05 v63.5,49.05
N$109  (via drill 0.35)
  Top 0.152: v20.32,43.82 19.68,43.18 14.61,43.18 13.97,42.55 IC45.6 | IC44.6 v27.94,42.86 | v66.04,45.72 IC42.11
  Route2 0.152: v27.94,42.86 26.99,43.82 v20.32,43.82
  Route3 0.152: v66.04,45.72 56.52,45.72 55.56,44.77 45.24,44.77 43.97,43.5 40.16,43.5 38.58,45.09 33.97,45.09 31.75,42.86 v27.94,42.86
N$110  (via drill 0.35)
  Top 0.152: v52.07,49.53 IC41.12 | 65.41,48.9 v63.5,50.8 | IC42.12 64.77,48.58 65.09,48.9 65.41,48.9 | IC42.10 67.31,48.58 66.99,48.9 65.41,48.9
  Route2 0.152: v52.07,49.53 55.24,52.71 61.59,52.71 v63.5,50.8
N$111  (via drill 0.35)
  Top 0.152: v43.18,44.45 42.55,44.45 40.64,42.55 IC43.5 | v55.24,45.72 55.24,46.36 54.61,46.99 IC41.10
  Route2 0.152: v43.18,44.45 43.79,45.06 54.59,45.06 v55.24,45.72
N$112
  Top 0.152: IC41.11 53.34,48.9 52.86,49.37 52.86,50.32 52.39,50.8 50.8,50.8 41.91,41.91 IC43.6
N$113  (via drill 0.35)
  Top 0.152: v24.13,42.86 IC44.3 24.13,40.01 24.45,39.69 26.35,39.69 26.67,40.01 IC44.5 | v12.7,42.86 IC45.5
  Route2 0.152: v24.13,42.86 v12.7,42.86
N$114
  Top 0.152: IC45.13 8.89,45.97 10.73,44.13 16.19,44.13 21.27,49.21 22.54,49.21 22.86,48.9 IC44.13 22.86,45.4 25.4,42.86 IC44.4
N$115  (via drill 0.35)
  Top 0.152: v11.43,42.86 IC45.4 | IC43.9 v41.91,49.05
  Route2 0.152: v11.43,42.86 13.02,44.45 20.02,44.45 20.05,44.47 27.62,44.47 27.67,44.43 28.21,44.43 28.23,44.45 35.24,44.45 38.26,47.47 40.32,47.47 v41.91,49.05
N$116  (via drill 0.35)
  Top 0.152: v10.16,39.37 IC45.3 | IC43.8 v43.18,49.05
  Route2 0.152: v10.16,39.37 8,41.53 8,45.15 11.75,48.9 12.86,50.01 12.86,50.8 12.86,50.96 14.13,52.23 42.39,52.23 43.18,51.44 v43.18,49.05
N$117  (via drill 0.35)
  Top 0.152: v10.16,49.53 IC45.12 | 24.13,50.48 25.72,50.48 26.67,49.53 IC44.10 | 24.13,50.48 21.43,50.48 v21.11,50.8 | 24.13,50.48 IC44.12
  Bottom 0.152: v10.16,49.53 10.48,49.21 19.53,49.21 v21.11,50.8
N$118  (via drill 0.35)
  Top 0.152: v16.19,45.72 16.19,45.4 15.56,44.77 13.65,44.77 12.7,45.72 IC45.10 | IC43.12 v38.1,48.9
  Route2 0.152: v16.19,45.72 19.21,45.72 20.64,47.15 23.18,47.15 24.61,45.72 27.64,45.72 27.67,45.74 28.21,45.74 28.23,45.72 34.92,45.72 v38.1,48.9
N$119  (via drill 0.35)
  Top 0.152: IC45.11 v11.43,46.04 | IC43.13 v36.83,49.05
  Route2 0.152: v11.43,46.04 12.38,46.04 14.61,48.26 16.19,48.26 16.67,48.74 19.53,48.74 24.13,48.74 25.08,49.69 31.11,49.69 32.54,48.26 36.04,48.26 v36.83,49.05
N$120  (via drill 0.35)
  Top 0.152: v52.07,92.71 IC50.11 | v123.19,76.2 124.46,77.47 IC53.3
  Route14 0.152: v123.19,76.2 120.02,79.38 120.02,80.64 117.87,82.79 116.6,82.79 107.31,92.08 99.54,92.08 98.74,91.28 96.68,91.28 95.89,92.08 55.56,92.08 54.45,90.96 53.82,90.96 v52.07,92.71
N$121  (via drill 0.35)
  Top 0.152: IC51.11 96.52,70.48 97.16,71.12 102.87,71.12 v107.95,76.2 | v115.25,82.23 117.79,82.23 120.23,79.79 122.87,79.79 123.19,79.48 IC53.2
  Route2 0.152: v107.95,76.2 109.22,76.2 v115.25,82.23
N$122  (via drill 0.35)
  Top 0.152: v20.64,75.88 13.02,75.88 11.43,77.47 IC48.11 | v125.73,76.2 127,77.47 IC53.5
  Route3 0.152: v20.64,75.88 36.83,92.08 50.64,92.08 51.75,90.96 54.45,90.96 55.56,92.08 95.89,92.08 96.68,91.28 98.74,91.28 99.54,92.08 118.11,92.08 125.73,84.45 v125.73,76.2
N$123  (via drill 0.35)
  Top 0.152: IC49.10 53.34,80.01 56.52,83.19 57.78,83.19 v59.69,85.09 | v118.75,90.17 121.92,90.17 125.73,86.36 IC53.11
  Route3 0.152: v59.69,85.09 77.95,85.09 78.58,85.73 81.12,85.73 81.76,85.09 113.67,85.09 v118.75,90.17
N$124  (via drill 0.35)
  Top 0.152: v53.34,92.71 IC50.10 | v63.98,95.73 117.63,95.73 127,86.36 IC53.10
  Bottom 0.152: v53.34,92.71 60.96,92.71 v63.98,95.73
N$125  (via drill 0.35)
  Top 0.152: IC51.10 97.79,70.38 98.02,70.61 103.63,70.61 v106.05,73.03 | IC53.9 v128.27,81.28
  Route2 0.152: v128.27,81.28 125.25,78.26 115.73,78.26 113.05,75.59 111.49,75.59 111.47,75.56 108.58,75.56 v106.05,73.03
N$126  (via drill 0.35)
  Top 0.152: v22.86,76.2 22.23,76.84 13.97,76.84 12.7,78.11 IC48.10 | v123.83,82.55 124.46,83.19 IC53.12
  Route3 0.152: v22.86,76.2 42.55,76.2 48.42,82.07 50.01,82.07 51.51,83.58 65.8,83.58 66.04,83.82 78.42,83.82 78.7,84.1 81.48,84.1 81.76,83.82 117,83.82 118.9,81.92 123.19,81.92 v123.83,82.55
N$127  (via drill 0.35)
  Top 0.152: IC9.9 67.31,91.44 v69.85,93.98 | v125.73,74.3 IC52.11
  Route15 0.152: v119.06,83.19 119.06,78.42 123.19,74.3 v125.73,74.3
  Bottom 0.152: v69.85,93.98 112.39,93.98 119.06,87.31 v119.06,83.19
N$128  (via drill 0.35)
  Top 0.152: v76.2,90.17 68.58,90.17 IC9.8 | IC52.10 v127,74.3
  Route2 0.152: v76.2,90.17 80.8,90.17 81.6,90.96 87.31,90.96 88.74,89.53 90.17,89.53 90.81,90.17 97.79,90.17 104.14,83.82 117,83.82 119.22,81.6 125.41,81.6 126.52,82.71 128.11,82.71 129.38,81.44 129.38,79.22 127,76.84 v127,74.3
N$129  (via drill 0.35)
  Top 0.152: v67.31,86.52 IC9.6 | v133.35,69.22 133.19,69.06 126.84,69.06 125.73,67.95 IC52.4
  Route2 0.152: v67.31,86.52 71.28,86.52 78.74,93.98 119.38,93.98 133.35,80.01 v133.35,69.22
N$130  (via drill 0.35)
  Top 0.152: IC9.5 66.04,83.19 66.67,82.55 v67.31,82.55 | IC52.3 v124.46,65.41
  Route14 0.152: v67.31,82.55 73.74,88.98 76.28,88.98 78.11,90.81 87.63,90.81 88.5,89.93 102.61,89.93 114.75,77.79 116.2,77.79 117.16,76.84 117.16,75.72 115.57,74.14 115.57,72.39 120.97,66.99 122.87,66.99 v124.46,65.41
N$131
  Top 0.152: IC9.13 62.23,91.44 62.87,92.08 65.41,92.08 66.04,91.44 IC9.10
N$132
  Top 0.152: IC9.4 64.77,87.31 63.5,88.58 IC9.12
N$133  (via drill 0.35)
  Top 0.152: v52.07,82.55 IC50.4 | IC54.3 95.28,73.1 v95.28,71.75
  Route3 0.152: v52.07,82.55 61.28,82.55 61.87,81.95 63.17,81.95 63.23,81.89 63.77,81.89 63.8,81.92 65.25,81.92 66.67,83.34 78.9,83.34 79.02,83.46 81.16,83.46 81.44,83.19 91.44,83.19 v93.34,81.28
  Route15 0.152: v95.28,71.75 95.28,79.35 v93.34,81.28
N$134  (via drill 0.35)
  Top 0.152: v96.52,74.61 IC54.4 | IC49.4 v52.07,71.75
  Route3 0.152: v66.04,77.47 81.92,77.47 82.87,76.52 94.61,76.52 v96.52,74.61
  Route15 0.152: v52.07,71.75 55.88,71.75 61.59,77.47 v66.04,77.47
N$135  (via drill 0.35)
  Top 0.152: IC48.4 11.43,74.93 v8.89,77.47 | v97.79,74.45 IC54.5
  Route2 0.152: v8.89,77.47 20.32,88.9 47.31,88.9 48.42,90.01 56.2,90.01 59.85,86.36 60.96,86.36 63.98,83.34 71.6,83.34 81.76,73.18 96.36,73.18 97.63,74.45 v97.79,74.45
N$136  (via drill 0.35)
  Top 0.152: IC51.4 v96.52,64.77 | IC54.2 93.98,71.85 v93.97,71.84
  Route2 0.152: v91.76,67.15 94.14,67.15 v96.52,64.77
  Route3 0.152: v93.97,71.84 91.76,69.63 v91.76,67.15
N$137  (via drill 0.35)
  Top 0.152: v50.8,81.6 IC50.3 | v98.42,77.47 97.79,78.11 IC54.10
  Route3 0.152: v50.8,81.6 62.55,81.6 65.09,79.06 81.6,79.06 82.07,79.53 85.41,79.53 86.2,78.74 97.16,78.74 v98.42,77.47
N$138  (via drill 0.35)
  Top 0.152: IC54.11 v96.52,77.47 | v50.8,74.61 IC49.3
  Route3 0.152: v50.8,74.61 61.75,74.61 65.56,78.42 82.07,78.42 82.71,79.06 84.77,79.06 85.72,78.11 95.89,78.11 v96.52,77.47
N$139  (via drill 0.35)
  Top 0.152: v95.25,61.47 IC51.3 | v99.19,81.28 99.06,81.15 IC54.9
  Route14 0.152: v99.19,81.28 96.39,81.28 91.69,76.58 91.69,74.45 92.7,73.45 95.47,73.45 96.41,72.5 96.41,71.32 95.89,70.8 v94.93,70.8
  Bottom 0.152: v95.25,61.47 95.25,62.87 93.82,64.29 93.82,69.69 v94.93,70.8
N$140  (via drill 0.35)
  Top 0.152: IC48.3 10.16,74.93 v7.62,77.47 | IC54.12 v95.25,81.28
  Route14 0.152: v95.25,81.28 94.61,81.28 93.34,82.55 v93.34,87
  Route15 0.152: v93.34,87 91.44,88.9 v90.81,88.9
  Bottom 0.152: v7.62,77.47 22.23,92.08 50.64,92.08 51.75,90.96 54.45,90.96 55.56,92.08 85.72,92.08 88.9,88.9 v90.81,88.9
N$141  (via drill 0.35)
  Top 0.152: v125.73,29.21 124.46,30.48 IC64.12
  Route14 0.152: v125.73,29.21 125.73,25.4 143.51,7.62 146.05,7.62 BEFEHL.4
N$142  (via drill 0.35)
  Top 0.152: IC55.2 139.7,32.38 v139.06,33.02 | v139.7,74.3 IC59.2 | v123.19,49.85 IC61.2 | v139.7,54.13 IC57.2 | IC58.2 139.7,64.27 v139.67,64.29 | v139.7,44.45 IC56.2 | IC62.2 v123.19,55.25 | IC60.2 v139.7,83.19 | IC4.6 v144.15,18.41
  Route2 0.152: v139.7,54.13 135.41,49.85 131.29,49.85 130.65,50.48 126.84,50.48 126.21,49.85 v123.19,49.85 v123.19,55.25
  Route3 0.152: v139.7,83.19 139.7,81.92 137.79,80.01 137.79,77.79 139.7,75.88 v139.7,74.3 140.97,73.03 140.97,65.59 v139.67,64.29
  Route14 0.152: v139.7,44.45 139.7,43.5 137.48,41.28 137.48,34.61 v139.06,33.02
  Route15 0.152: v144.15,18.41 144.15,19.21 138.91,24.45 138.91,32.86 v139.06,33.02 | v139.67,64.29 139.67,58.93 138.62,57.88 138.62,55.22 v139.7,54.13
  Bottom 0.152: v139.7,44.45 139.7,46.04 140.81,47.15 140.81,53.02 v139.7,54.13
N$143
  Top 0.152: IC64.8 129.54,26.67 133.99,22.22 133.99,17.14 BEFEHL.3
N$144  (via drill 0.35)
  Top 0.152: IC4.10 v145.41,27.3 | IC59.3 140.97,72.07 142.24,70.8 v144.15,70.8 | IC59.10 143.51,77.47 v145.41,75.56 | v124.46,47.94 IC61.3 | IC55.3 140.97,32.38 v140.34,33.02 | IC57.3 140.97,52.07 v139.7,50.8 | IC57.10 143.51,57.79 v144.15,57.15 | v145.41,40.32 143.51,38.42 IC55.10 143.51,36.04 v144.94,34.61 | v128.11,48.26 127,49.37 IC61.10
  Route2 0.152: v128.11,48.26 127.48,48.26 127.16,47.94 v124.46,47.94 | v144.15,57.15 144.15,55.25 v139.7,50.8 | v145.41,27.3 145.41,32.7 144.94,33.18 v144.94,34.61
  Route14 0.152: v145.41,75.56 145.41,72.07 v144.15,70.8
  Bottom 0.152: 134.62,45.72 132.24,48.1 128.27,48.1 v128.11,48.26 | 134.62,45.72 v139.7,50.8 | v145.41,40.32 145.41,45.56 145.69,45.84 145.69,48.77 145.41,49.05 145.41,55.88 v144.15,57.15 144.15,65.72 145.91,67.49 145.91,69.03 v144.15,70.8 | 134.62,45.72 140.81,39.53 140.81,38.42 138.43,36.04 138.43,34.92 v140.34,33.02
N$145  (via drill 0.35)
  Top 0.152: v127,22.86 IC64.5
  Bottom 0.152: v127,22.86 125.57,21.43 125.57,20.48 128.27,17.78 140.97,17.78 142.24,16.51 BEFEHL.2
N$146  (via drill 0.35)
  Top 0.152: v144.62,86.36 144.62,86.52 142.24,88.9 IC60.11 | v142.24,86.36 IC60.4 142.24,82.23 141.6,81.6 141.6,81.28 142.24,80.64 IC59.11 IC59.4 | IC55.11 142.24,38.73 143.51,40.01 v143.51,40.16 | v142.88,27.94 IC4.12 | v142.24,29.84 IC55.4 142.24,32.52 v142.21,32.54 | IC56.4 v142.24,41.28 | IC56.11 v142.24,47.31
  Route2 0.152: v142.24,86.36 v144.62,86.36 | v142.88,27.94 142.88,29.21 v142.24,29.84
  Route3 0.152: v142.24,41.28 142.24,32.57 v142.21,32.54
  Route14 0.152: v142.24,29.84 143.19,29.84 143.51,30.16 v143.51,40.16 143.51,46.04 v142.24,47.31
  Bottom 0.152: v144.62,86.36 144.15,85.88 144.15,79.69 145.73,78.11 145.73,77.79 144.15,76.2 144.15,72.39 146.69,69.85 146.69,65.56 146.05,64.93 146.05,62.07 147.16,60.96 147.16,40.64 146.05,39.53 144.15,39.53 v143.51,40.16
N$147  (via drill 0.35)
  Top 0.152: IC64.1 121.92,22.86 v124.46,20.32
  Bottom 0.152: v124.46,20.32 127.64,17.14 138.91,17.14 140.97,15.08 140.97,7.62 BEFEHL.1
N$148  (via drill 0.35)
  Top 0.152: 140.97,55.88 143.51,53.34 IC57.5 143.51,50.8 143.19,50.48 141.29,50.48 140.97,50.16 IC56.12 140.97,46.99 143.51,44.45 IC56.5 143.51,41.28 140.97,38.73 IC55.12 140.97,35.88 143.51,33.34 IC55.5 143.51,29.69 142.4,28.57 140.34,28.57 139.06,27.3 IC4.15 | IC57.12 140.97,55.88 | 143.51,63 IC58.5 143.67,63.12 143.67,64.61 140.97,67.31 IC58.12 140.97,70.33 140.34,70.96 v139.54,70.96 | v140.02,55.72 140.18,55.88 140.97,55.88
  Bottom 0.152: v139.54,70.96 139.54,70.94 136.34,67.74 136.34,59.4 v140.02,55.72
N$149
  Top 0.152: IC64.13 IC64.2 123.19,22.86 127,19.05 | IC64.9 128.27,29.58 128.59,29.27 128.59,26.45 128.27,26.14 IC64.6 128.27,21.43 127,20.16 127,19.05 | 127,19.05 CHECK.1
N$150  (via drill 0.35)
  Top 0.152: IC65.12 110.49,26.67 v113.03,29.21 | v124.46,40.96 IC63.12
  Bottom 0.152: IN/NUMBER.4 137.16,7.78 130.02,14.92 127.32,14.92 v113.03,29.21 113.98,29.21 121.92,37.15 121.92,40.64 122.24,40.96 v124.46,40.96
N$151  (via drill 0.35)
  Top 0.152: v116.84,24.13 115.57,25.4 IC65.8 | IC63.8 v129.54,40.96
  Route3 0.152: v129.54,40.96 132.4,38.1 132.4,14.92 130.81,13.34 v128.91,13.34
  Bottom 0.152: IN/NUMBER.3 134.62,7.62 v128.91,13.34 127.79,13.34 117,24.13 v116.84,24.13
N$152  (via drill 0.35)
  Top 0.152: IC65.5 113.03,20.95 v113.67,21.59 | v127,33.02 IC63.5
  Route14 0.152: v127,33.02 115.57,21.59 v113.67,21.59
  Bottom 0.152: v113.67,21.59 117.47,21.59 132.08,6.98 IN/NUMBER.2
N$153  (via drill 0.35)
  Top 0.152: v107.95,17.78 IC65.1 | IC63.1 121.92,34.92 118.11,31.11 v118.11,17.78
  Route2 0.152: v107.95,17.78 v118.11,17.78 IN/NUMBER.1
N$154  (via drill 0.35)
  Top 0.152: v107.95,33.66 IC66.1 | IC63.13 v123.19,40.01 IC63.2 v123.19,34.61 | v128.27,34.92 IC63.6 128.27,40.34 128.29,40.37 128.29,40.91 128.27,40.94 IC63.9
  Route2 0.152: v123.19,34.61 123.51,34.92 v128.27,34.92
  Route14 0.152: v123.19,40.01 114.94,31.75 109.86,31.75 v107.95,33.66
N$155
  Top 0.152: IC68.5 113.03,53.34 112.87,53.5 113.03,53.66 113.03,54.29 112.71,54.61 111.12,54.61 110.49,53.98 IC68.3
N$156  (via drill 0.35)
  Top 0.152: IC67.3 v110.49,44.13 | v114.74,34.26 113.03,32.55 IC66.5
  Route14 0.152: v110.49,44.13 110.49,40.96 112.52,38.93 112.52,36.16 114.42,34.26 v114.74,34.26
N$158  (via drill 0.35)
  Top 0.152: IC67.4 v111.76,41.28 | v109.22,29.84 IC66.2
  Route15 0.152: v111.76,41.28 111.76,32.38 v109.22,29.84
N$159  (via drill 0.35)
  Top 0.152: IC65.9 114.3,24.5 114.62,24.19 114.62,21.21 114.3,20.9 IC65.6 114.3,19.05 109.54,14.29 99.38,14.29 | 109.22,24.13 IC65.13 v109.22,27.94 | 109.22,24.13 IC65.2 | R.1 84.14,14.29 99.38,14.29 | 109.22,24.13 99.38,14.29 | IC66.13 v109.22,35.88
  Route2 0.152: v109.22,27.94 109.22,28.35 110.46,29.59 110.46,30.73 108.74,32.45 108.74,35.4 v109.22,35.88
N$160  (via drill 0.35)
  Top 0.152: v114.3,39.05 IC66.9 | IC67.10 113.03,47.62 v115.57,45.09
  Bottom 0.152: v115.57,45.09 115.57,40.32 v114.3,39.05
N$161  (via drill 0.35)
  Top 0.152: v110.49,38.58 IC66.12 | IC67.11 v111.76,46.99
  Route2 0.152: v110.49,38.58 110.49,39.85 109.7,40.64 109.7,44.93 v111.76,46.99
N$167  (via drill 0.35)
  Top 0.152: IC47.1 92.08,80.96 90.49,79.38 90.49,66.36 v90.81,66.04
  Route14 0.152: v90.81,66.04 90.81,45.09 112.71,23.18 112.71,15.56 SAME.1
N$171  (via drill 0.35)
  Top 0.152: IC47.15 93.34,88.9 v93.98,88.27
  Route15 0.152: v93.98,88.27 97.16,88.27 105.09,80.33 105.09,76.84 109.06,72.87 112.55,72.87 130.1,55.32 131.52,55.32 132.08,54.77 132.08,13.97 CARRY.1
N$173  (via drill 0.35)
  Top 0.152: v92.71,22.22 IC70.1 | IC69.10 v113.03,67.63
  Route3 0.152: v92.71,22.22 92.71,22.86 105.57,35.72 105.57,55.4 106.84,56.67 106.84,59.21 109.54,61.91 109.54,64.45 112.71,67.63 v113.03,67.63
N$174  (via drill 0.35)
  Top 0.152: v93.98,20.32 IC70.2 | IC69.11 v111.76,64.77
  Route3 0.152: v93.98,20.32 93.66,20.64 93.66,20.98 93.32,21.32 93.32,21.86 93.66,22.2 93.66,23.18 107.08,36.59 107.08,39.29 109.7,41.91 109.7,45.24 110.49,46.04 110.49,48.26 109.54,49.21 109.54,56.2 112.55,59.21 112.55,63.98 v111.76,64.77
N/IN/N0  (via drill 0.35)
  Top 0.152: IC63.3 124.46,34.29 v123.83,33.66 | v78.74,67.79 IC8.13
  Route3 0.152: v106.05,57.47 v106.05,62.23
  Route15 0.152: v106.05,62.23 90.17,62.23 88.27,64.14 82.87,64.14 79.22,67.79 v78.74,67.79 | 120.65,33.66 120.65,36.83 106.68,50.8 106.68,51.75 106.05,52.39 v106.05,57.47 | 120.65,33.66 v123.83,33.66 | 120.65,5.68 120.65,33.66
N/IN/N1  (via drill 0.35)
  Top 0.152: v125.73,33.02 IC63.4 | v83.82,61.59 IC8.6
  Route3 0.152: v125.73,33.02 125.73,30.48 v106.68,11.43
  Route14 0.152: v83.82,61.59 83.82,58.42 87.63,54.61 87.63,51.59 88.9,50.32 88.9,47.62 88.27,46.99 88.27,30.48 97.39,21.35 97.39,15.64 101.6,11.43 v106.68,11.43
N/IN/N2  (via drill 0.35)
